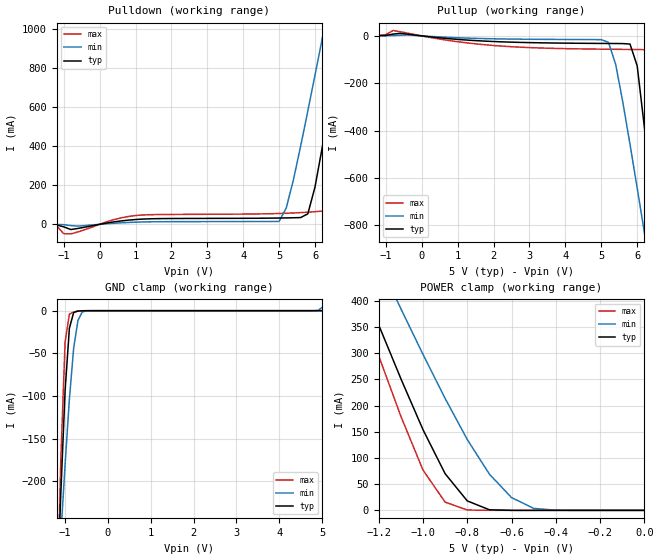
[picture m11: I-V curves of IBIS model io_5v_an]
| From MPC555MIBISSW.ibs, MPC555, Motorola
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| io_5v_an (5v ANALOG PAD)
[Model]   io_5v_an
Model_type   I/O
Polarity   Non-Inverting
|   typ   min   max
C_comp   4.7270e-13   4.1940e-13   5.4410e-13
| CAP models
| typical : model= typ
| maximum : model= wcs
| minimum : model= bcs
[Voltage range]   5.0v   4.5v   5.5v
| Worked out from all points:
|   slope of the pulldown table from 0 to 0.75 V, typ, clamps not added: 36.8 ohm
|   slope of the pullup table from 0 to 0.75 V, typ, clamps not added: 64.3 ohm
|   GND clamp passes 1 mA (typ) near -0.74 V on its own axis
|   POWER clamp passes 1 mA (typ) near -0.69 V on its own axis
|  typical: model = typ,  temp = 25,  vdd = 5.0
|  maximum: model = bcs,  temp = -40, vdd = 5.5
|  minimum: model = wcs,  temp = 150, vdd = 4.5
[Pulldown]
|  Voltage   I(typ)   I(min)   I(max)
-5V       -240uA     -80uA      -490uA
-1.4V     -1.679mA   -560uA     -3.107mA
-800mV    -26.75mA   -6.541mA   -48.84mA
1V        24.56mA    10.89mA    44.97mA
5V        32.25mA    14.78mA    55.47mA
5.2V      32.85mA    84.21mA    56.67mA
5.8V      53.76mA    581.1mA    62.16mA
6.2V      392.7mA    951.3mA    67.83mA
6.4V      606.4mA    1.139A     86.87mA
6.8V      1.046A     1.517A     494.6mA
7.2V      1.492A     1.899A     1A
10V       4.688A     4.599A     4.7A
[GND_clamp]
-5V       -6.286A    -4.003A    -9.278A
-1.2V     -352.4mA   -351.9mA   -373.6mA
-1.1V     -214.5mA   -264.1mA   -174.5mA
-1V       -93.75mA   -180.2mA   -36.84mA
-900mV    -20.64mA   -103.8mA   -4.008mA
-800mV    -2.016mA   -43.86mA   -1.601mA
-700mV    -441uA     -11.51mA   -530.8uA
-600mV    -100.9uA   -1.477mA   -71.46uA
-500mV    -12.89uA   -156.2uA   -2.911uA
4.8V      53.73pA    19.09uA    46.07pA
4.9V      56pA       287.6uA    48.18pA
5V        58.61pA    3.8mA      50.29pA
[Pullup]
-5V       180uA      114uA      247uA
-800mV    7.533mA    1.073mA    22.78mA
5.2V      -32.01mA   -27.24mA   -56.34mA
5.4V      -32.18mA   -119.6mA   -56.64mA
5.8V      -34.5mA    -457.9mA   -57.17mA
6V        -126.4mA   -642.2mA   -57.41mA
6.2V      -385.2mA   -829.7mA   -58.16mA
6.4V      -679mA     -1.019A    -61.85mA
6.6V      -982.4mA   -1.21A     -232.5mA
6.8V      -1.29A     -1.402A    -648.2mA
7V        -1.601A    -1.594A    -1.099A
10V       -6.322A    -4.507A    -8.158A
[POWER_clamp]
-5V       4.559A     4.065A     5.11A
-1.3V     459.2mA    564.9mA    415.1mA
-1.2V     354.1mA    474.5mA    295.2mA
-1.1V     251.6mA    385.3mA    179.8mA
-1V       154.2mA    298mA      77.05mA
-900mV    70.04mA    213.8mA    15.71mA
-800mV    18.08mA    135.3mA    606.6uA
-700mV    1.079mA    69.19mA    104.9uA
-600mV    34.26uA    24.39mA    21.06uA
-500mV    2.117uA    3.8mA      1.676uA
-400mV    134.1nA    287.6uA    45.9nA
0V        58.61pA    5.535nA    60.84pA
| RAMP models
| typical dv/dt : model=typ, temp=25
| maximum dv/dt : model=bcs, temp=-40
| minimum dv/dt : model=wcs, temp=150
|		 typ   min   max
[Ramp]
dV/dt_r   0.901647/4.3306E-09   0.452668/4.35217E-09   3.34206/3.86435E-09
dV/dt_f   0.901647/4.35724E-09   0.452668/3.86823E-09   3.34206/4.08917E-09
